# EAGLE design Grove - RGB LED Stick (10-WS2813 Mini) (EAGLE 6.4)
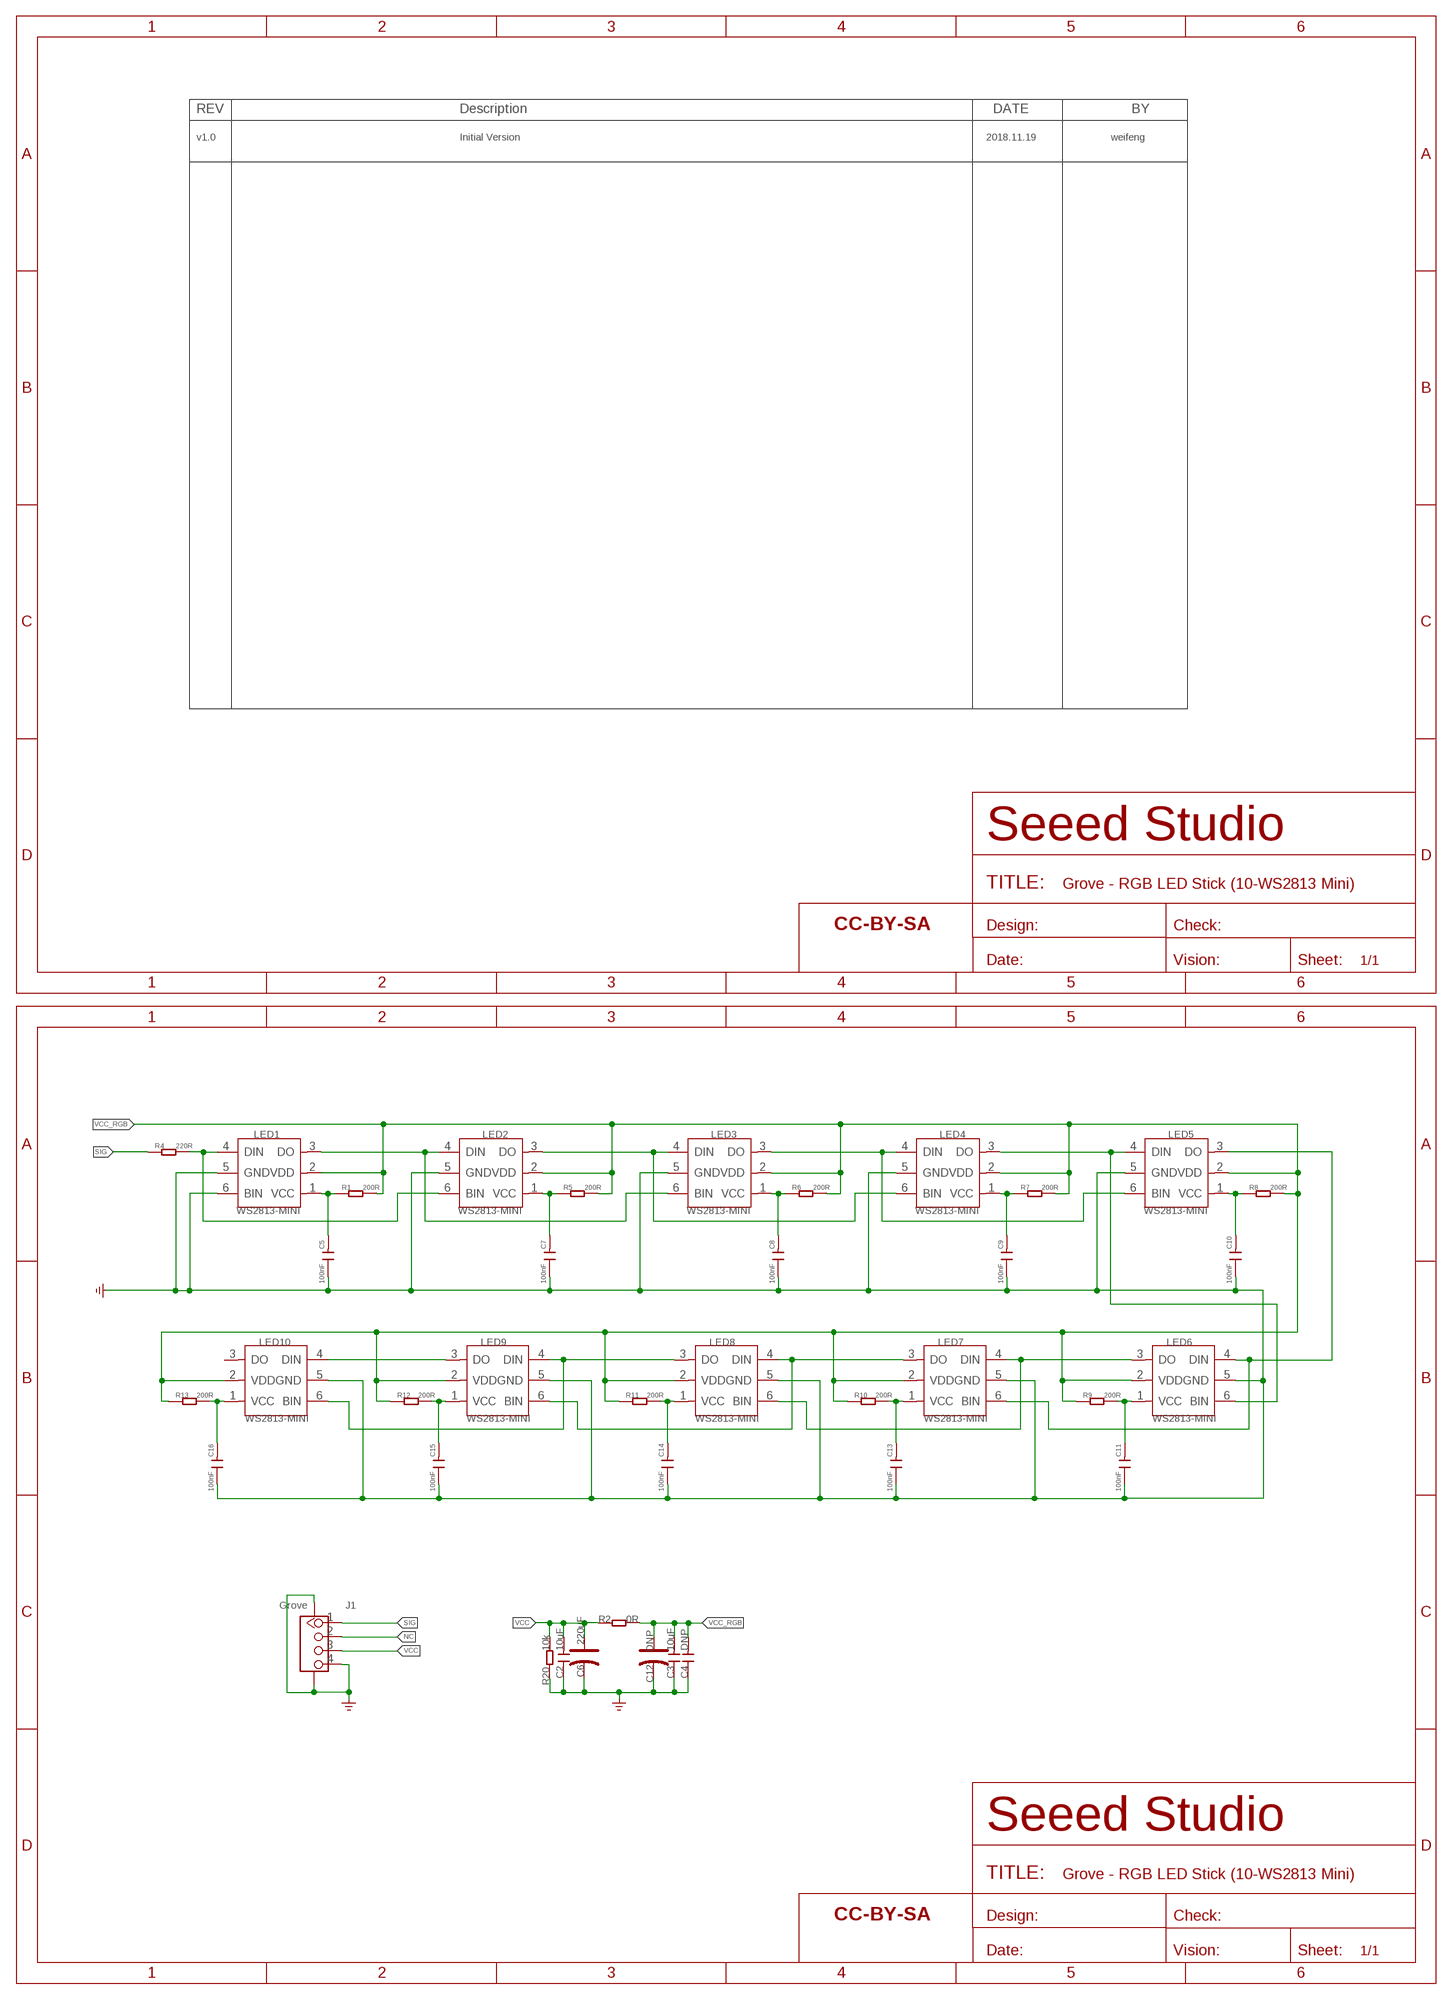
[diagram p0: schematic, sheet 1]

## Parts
C2  10uF  CAP-0805  [C0805]
C3  10uF  CAP-0805  [C0805]
C4  DNP  CAP-0603  [C0603]
C5  100nF  C-0603  [C0603]
C6  220uF  CAP-POLAR-AVX-B  [AVX-B]
C7  100nF  C-0603  [C0603]
C8  100nF  C-0603  [C0603]
C9  100nF  C-0603  [C0603]
C10  100nF  C-0603  [C0603]
C11  100nF  C-0603  [C0603]
C12  DNP  CAP-POLAR-AVX-B  [AVX-B]
C13  100nF  C-0603  [C0603]
C14  100nF  C-0603  [C0603]
C15  100nF  C-0603  [C0603]
C16  100nF  C-0603  [C0603]
FR1  SEEEDSTUDIO-OPEN-SCH-FRAME  [SEEEDSTUDIO-PCB-FRAME]
FR2  SEEEDSTUDIO-OPEN-SCH-FRAME  [SEEEDSTUDIO-PCB-FRAME]
J1  Grove  GROVE-CONNECTOR-SMD'DD'  [HW4-SMD-2.0]
LED1  WS2813-MINI  LED-RGB-6P-WS2813  [LED6-1.1-3.5X3.5X0.95MM]
LED2  WS2813-MINI  LED-RGB-6P-WS2813  [LED6-1.1-3.5X3.5X0.95MM]
LED3  WS2813-MINI  LED-RGB-6P-WS2813  [LED6-1.1-3.5X3.5X0.95MM]
LED4  WS2813-MINI  LED-RGB-6P-WS2813  [LED6-1.1-3.5X3.5X0.95MM]
LED5  WS2813-MINI  LED-RGB-6P-WS2813  [LED6-1.1-3.5X3.5X0.95MM]
LED6  WS2813-MINI  LED-RGB-6P-WS2813  [LED6-1.1-3.5X3.5X0.95MM]
LED7  WS2813-MINI  LED-RGB-6P-WS2813  [LED6-1.1-3.5X3.5X0.95MM]
LED8  WS2813-MINI  LED-RGB-6P-WS2813  [LED6-1.1-3.5X3.5X0.95MM]
LED9  WS2813-MINI  LED-RGB-6P-WS2813  [LED6-1.1-3.5X3.5X0.95MM]
LED10  WS2813-MINI  LED-RGB-6P-WS2813  [LED6-1.1-3.5X3.5X0.95MM]
R1  200R  R-0603  [R0603]
R2  0R  RES-0805  [R0805]
R4  220R  R-0603  [R0603]
R5  200R  R-0603  [R0603]
R6  200R  R-0603  [R0603]
R7  200R  R-0603  [R0603]
R8  200R  R-0603  [R0603]
R9  200R  R-0603  [R0603]
R10  200R  R-0603  [R0603]
R11  200R  R-0603  [R0603]
R12  200R  R-0603  [R0603]
R13  200R  R-0603  [R0603]
R20  10k  RES-0603  [R0603]

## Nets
GND: C2.1 C3.1 C4.1 C5.1 C6.- C7.1 C8.1 C9.1 C10.1 C11.1 C12.- C13.1 C14.1 C15.1 C16.1 J1.4 J1.SS1 J1.SS2 LED1.5(GND) LED1.6(BIN) LED2.5(GND) LED3.5(GND) LED4.5(GND) LED5.5(GND) LED6.5(GND) LED7.5(GND) LED8.5(GND) LED9.5(GND) LED10.5(GND) R20.1 ; supply symbol labelled GND_POWER
N$1: C5.2 LED1.1(VCC) R1.1
N$2: LED2.3(DO) LED3.4(DIN) LED4.6(BIN)
N$3: C9.2 LED4.1(VCC) R7.1
N$5: LED3.3(DO) LED4.4(DIN) LED5.6(BIN)
N$6: LED1.4(DIN) LED2.6(BIN) R4.2
N$7: LED4.3(DO) LED5.4(DIN) LED6.6(BIN)
N$8: C10.2 LED5.1(VCC) R8.1
N$9: LED5.3(DO) LED6.4(DIN) LED7.6(BIN)
N$10: C7.2 LED2.1(VCC) R5.1
N$12: C11.2 LED6.1(VCC) R9.2
N$14: LED1.3(DO) LED2.4(DIN) LED3.6(BIN)
N$16: C8.2 LED3.1(VCC) R6.1
N$18: LED6.3(DO) LED7.4(DIN) LED8.6(BIN)
N$21: C13.2 LED7.1(VCC) R10.2
N$23: LED7.3(DO) LED8.4(DIN) LED9.6(BIN)
N$26: C14.2 LED8.1(VCC) R11.2
N$29: LED8.3(DO) LED9.4(DIN) LED10.6(BIN)
N$32: C15.2 LED9.1(VCC) R12.2
N$35: LED9.3(DO) LED10.4(DIN)
N$38: C16.2 LED10.1(VCC) R13.2
NC: J1.2
SIG: J1.1 R4.1
VCC: C2.2 C6.+ J1.3 R2.1 R20.2
VCC_RGB: C3.2 C4.2 C12.+ LED1.2(VDD) LED2.2(VDD) LED3.2(VDD) LED4.2(VDD) LED5.2(VDD) LED6.2(VDD) LED7.2(VDD) LED8.2(VDD) LED9.2(VDD) LED10.2(VDD) R1.2 R2.2 R5.2 R6.2 R7.2 R8.2 R9.1 R10.1 R11.1 R12.1 R13.1
Unconnected: LED10.3(DO)

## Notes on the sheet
- v1.0 | Initial Version | 2018.11.19 | weifeng

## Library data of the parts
C2-C4 = Discrete-new:CAP: Ceramic Capacitors
C5 C7-C11 C13-C16 = Discrete-small:C*: Ceramic Capacitors
C6 C12 = Discrete-new:CAP-POLAR: Electrolytic Capacitors,Tantalum Capacitors and Super Capacitors
FR1 FR2 = moudle-new:SEEEDSTUDIO-OPEN-SCH-FRAME
J1 = Connector-new:GROVE-CONNECTOR-SMD: 4P-SMD-2.0:320110030;4P-SMD-2.0-90D:320110032
LED1-LED10 = Discrete-new:LED-RGB-6P
R1 R4-R13 = Discrete-small:R*
R2 R20 = Discrete-new:RES

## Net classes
3 usbvcc: width 0.203 mm, drill 0.305 mm, clearance 0.203 mm

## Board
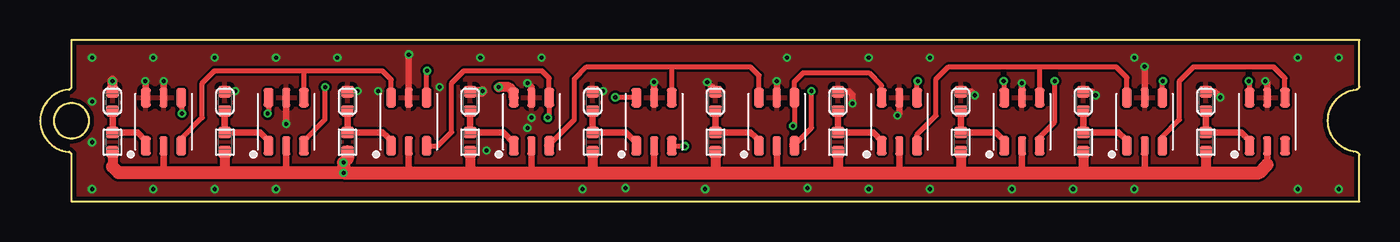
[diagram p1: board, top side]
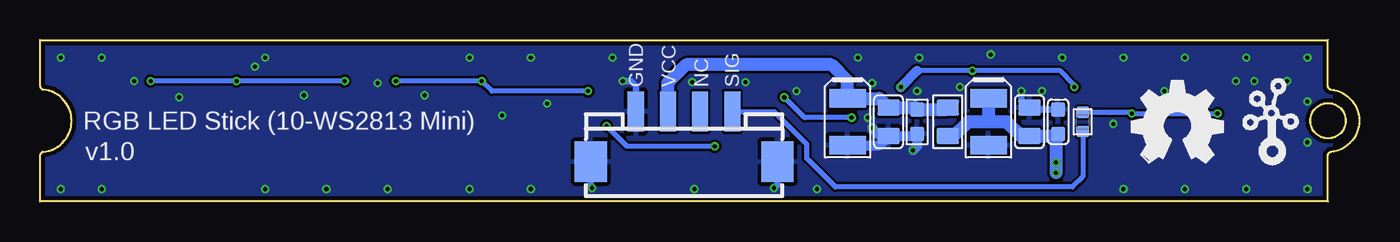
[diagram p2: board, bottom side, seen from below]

Size 81.96 x 10.03 mm. Coordinates in mm from the lower left corner, seen from the top.
Outline: 81.96,0 81.96,2.88 arc85 81.78,3.07 arc-169 81.78,6.96 arc85 81.96,7.16 81.96,10.03 1.95,10.03 1.95,7.16 arc-85 1.77,6.96 arc169 1.77,3.07 arc-85 1.95,2.88 1.95,0 81.96,0
Outline: 1.94,3.92 arc180 1.94,6.12 arc180 1.94,3.92
Copper layers (1*16): Top 0.035mm / dielectric 1.5mm / Bottom 0.035mm
Design rules "SeeedStudio_2layer_DRU_no_angle_20140221": minimum track width 1mil, minimum drill 10mil, track to track 6mil, track to pad 6mil, pad to pad 6mil, via to via 6mil, smd to smd 0mil, copper to edge 10mil, drill to drill 10mil, minimum pad ring 4mil, minimum via ring 4mil, stop-mask expansion 2mil, vias tented up to drill 25mil, thermal gap 10mil

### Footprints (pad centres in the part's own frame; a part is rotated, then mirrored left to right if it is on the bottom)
C0805 = smd 1.016 x 1.397: 1 -0.889,0; 2 0.889,0
C0603 = smd 0.889 x 0.889: 1 -0.762,0; 2 0.762,0
C0603' = smd 0.762 x 0.696: 1 0,0.602; 2 0,-0.602
AVX-B = smd 1.143 x 2.286: + 1.46,0; - -1.46,0
HW4-SMD-2.0 = smd 1 x 2.5: 1 -3,0; 2 -1,0; 3 1,0; 4 3,0 | smd 2 x 2.5: SS1 -5.8,3.123; SS2 5.8,3.123
LED6-1.1-3.5X3.5X0.95MM = smd 1.2 x 0.6: 1 -1.5,1.1; 3 -1.5,-1.1; 4 1.5,-1.1; 6 1.5,1.1 | smd 1.2 x 0.5: 2 -1.5,0; 5 1.5,0
R0603 = smd 0.762 x 0.696: 1 0,0.602; 2 0,-0.602
R0805 = smd 1.016 x 1.397: 1 -0.889,0; 2 0.889,0
R0603' = smd 0.889 x 0.889: 1 -0.762,0; 2 0.762,0

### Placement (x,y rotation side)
C2  29.25,4.95 90 bottom
C3  20.49,4.95 270 bottom
C4  18.71,4.95 270 bottom
C5  100nF  [C0603']  4.49,6.22 0 top
C6  31.79,4.95 90 bottom
C7  100nF  [C0603']  11.47,6.22 0 top
C8  100nF  [C0603']  19.09,6.22 0 top
C9  100nF  [C0603']  26.71,6.22 0 top
C10  100nF  [C0603']  34.33,6.22 0 top
C11  100nF  [C0603']  41.95,6.22 0 top
C12  23.03,4.95 90 bottom
C13  100nF  [C0603']  49.57,6.22 0 top
C14  100nF  [C0603']  57.19,6.22 0 top
C15  100nF  [C0603']  64.81,6.22 0 top
C16  100nF  [C0603']  72.43,6.22 0 top
FR1  not placed on the board
FR2  not placed on the board
J1  41.95,5.59 180 bottom
LED1  7.66,4.95 90 top
LED2  15.28,4.95 90 top
LED3  22.9,4.95 90 top
LED4  30.52,4.95 90 top
LED5  38.14,4.95 90 top
LED6  45.76,4.95 90 top
LED7  53.38,4.95 90 top
LED8  61,4.95 90 top
LED9  68.62,4.95 90 top
LED10  76.24,4.95 90 top
R1  4.49,3.68 0 top
R2  25.57,4.95 270 bottom
R4  17.19,4.95 180 bottom
R5  11.47,3.68 0 top
R6  19.09,3.68 0 top
R7  26.71,3.68 0 top
R8  34.33,3.68 0 top
R9  41.95,3.68 180 top
R10  49.57,3.68 180 top
R11  57.19,3.68 180 top
R12  64.81,3.68 180 top
R13  72.43,3.68 180 top
R20  10k  [R0603']  27.48,4.95 90 bottom
U$7  [GROVE-SILK-SMALL]  7.64,2.13 0 bottom
U$8  [OSHW_FILLX200_NOTEXT]  14.14,2.41 0 bottom

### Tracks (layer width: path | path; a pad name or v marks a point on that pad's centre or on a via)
GND  (via drill 0.25 pad 0.51)
  Top 0.406: LED1.5 v7.66,7.49 | LED1.6 6.56,7.45 v6.52,7.49 | C7.1 12.08,6.82 v12.11,6.86 | LED2.5 v15.28,4.83 | C8.1 19.7,6.82 v19.73,6.86 | LED3.5 v22.9,9.14 | LED4.5 30.52,7.11 v30.27,7.37 | C10.1 34.94,6.82 v34.97,6.86 | LED5.5 v38.14,7.43 | C11.1 41.95,6.92 v41.45,7.43 | LED6.5 v45.76,7.49 | C13.1 50.24,6.82 50.46,6.6 v50.46,6.1 | C14.1 57.86,6.82 v58.08,6.6 | LED8.5 v61,7.37 | C15.1 65.35,6.82 v65.58,6.6 | LED9.5 v68.62,8.38 | C16.1 72.97,6.82 v73.32,6.48 | LED10.5 76.24,7.37 v76.12,7.49 | LED7.5 53.38,5.46 v53.26,5.33
  Top 0.61: C5.1 v4.49,7.49 | C9.1 27.44,6.82 v27.48,6.86
  Bottom 0.406: v21,6.86 21,6.35 C3.1 20.36,5.71 C4.1 | J1.SS1 36.15,1.04 v36.37,0.82 | J1.SS2 47.75,0.91 v47.67,0.82 | J1.4 44.95,7.19 45.26,7.49 v45.76,7.49
  Bottom 0.61: v27.73,3.17 27.48,3.43 R20.1 27.6,4.06 C2.1 | C2.1 29.76,4.06 v30.27,4.57 | C6.- 29.82,3.49 C2.1
  other vias: 3.22,8.95 3.22,6.22 3.22,3.68 3.22,0.76 7.03,0.76 10.84,0.76 7.03,8.95 10.84,8.95 14.65,8.95 18.46,8.95 14.65,0.76 33.7,0.76 27.35,8.95 31.16,8.95 41.32,0.76 46.4,8.95 51.48,0.76 51.48,8.95 55.29,8.95 55.29,0.76 67.99,8.95 67.99,0.76 64.18,0.76 60.37,0.76 78.15,8.95 78.15,0.76 80.69,0.76 80.69,8.95 30.52,5.21 24.81,7.11
  pour Bottom (isolate 0.152): 1.31,10.67 82.59,10.67 82.59,-0.76 3.22,-0.76 3.22,-1.4 1.31,-1.4
  pour Top (isolate 0.152): 1.31,10.67 82.59,10.67 82.59,-0.76 1.31,-0.76
N$1
  Top 0.406: LED1.1 6.56,3.77 6.05,4.28 R1.1 C5.2
N$2  (via drill 0.25 pad 0.51)
  Top 0.305: LED3.4 24,8.08 v24.05,8.13 | LED2.3 16.38,3.77 17.7,5.08 v17.7,7.11
  Top 0.61: LED4.6 29.42,6.81 29.13,7.11 v28.49,7.11
  Bottom 0.305: v17.7,7.11 17.7,7.24 18.59,8.13 v24.05,8.13 27.48,8.13
  Bottom 0.61: 27.48,8.13 v28.49,7.11
N$3
  Top 0.406: C9.2 R7.1 28.78,4.28 29.42,3.64 LED4.1
N$5  (via drill 0.25 pad 0.51)
  Top 0.305: v31.54,5.21 31.62,5.29 LED4.4 31.62,7.66 31.16,8.13 26.33,8.13 25.57,7.37 25.57,4.32 24.71,3.45 LED3.3 | LED5.6 35.75,6.45 v35.73,6.48
  Bottom 0.305: v31.54,5.21 34.46,5.21 v35.73,6.48
N$6  (via drill 0.25 pad 0.51)
  Top 0.305: LED2.6 14.18,5.5 v14.14,5.46 | v8.81,5.46 8.81,6.41 LED1.4
  Bottom 0.305: v8.81,5.46 v14.14,5.46 14.23,5.55 R4.2
N$7
  Top 0.305: 39.29,8.38 33.95,8.38 33.19,7.62 33.19,5.08 31.62,3.51 | 39.29,8.38 44.11,8.38 44.66,7.83 LED6.6 | LED5.4 39.24,8.34 39.29,8.38
  Top 0.61: LED4.3 31.62,3.51
N$8
  Top 0.406: C10.2 R8.1 36.4,4.28 37.04,3.64 LED5.1
N$9  (via drill 0.25 pad 0.51)
  Top 0.305: LED5.3 40.02,3.45 v40.05,3.43 | v46.78,4.7 46.86,4.78 LED6.4 46.86,7.45 47.41,8 51.48,8 52.28,7.2 LED7.6
  Bottom 0.305: v40.05,3.43 45.51,3.43 v46.78,4.7
N$10
  Top 0.406: C7.2 R5.1 13.67,4.28 14.08,3.87 14.14,3.81 14.18,3.77 LED2.1
N$12
  Top 0.406: C11.2 R9.2 44.15,4.28 44.43,4 44.49,3.94 44.66,3.77 LED6.1
N$14
  Top 0.305: LED1.3 8.76,3.89 10.08,5.21 10.08,7.37 10.84,8.13 16.3,8.13 | 16.3,8.13 21.25,8.13 21.8,7.58 LED3.6 | LED2.4 16.38,8.04 16.3,8.13
N$16
  Top 0.406: C8.2 R6.1 21.29,4.28 21.57,4 21.63,3.94 21.8,3.77 LED3.1
N$18  (via drill 0.25 pad 0.51)
  Top 0.305: 46.86,3.51 47.92,4.57 v47.92,6.86 | LED7.4 54.48,7.45 v54.53,7.49 | LED8.6 59.9,7.45 v59.86,7.49
  Top 0.61: LED6.3 46.86,3.51
  Bottom 0.305: v47.92,6.86 53.89,6.86 v54.53,7.49 v59.86,7.49
N$21
  Top 0.406: C13.2 R10.2 51.77,4.28 52.28,3.77 LED7.1
N$23
  Top 0.305: LED7.3 54.48,4.15 55.67,5.33 55.67,7.62 56.43,8.38 62.02,8.38 | 62.02,8.38 66.85,8.38 67.52,7.7 LED9.6 | LED8.4 62.1,8.3 62.02,8.38
N$26
  Top 0.406: C14.2 R11.2 59.39,4.28 59.9,3.77 LED8.1
N$29  (via drill 0.25 pad 0.51)
  Top 0.305: LED8.3 62.1,4.02 63.04,4.95 v63.04,7.49 | LED9.4 69.72,7.45 v69.77,7.49 | LED10.6 75.14,7.45 v75.1,7.49
  Bottom 0.305: v63.04,7.49 v69.77,7.49 v75.1,7.49
N$32
  Top 0.406: C15.2 R12.2 67.01,4.28 67.42,3.87 67.48,3.81 67.52,3.77 LED9.1
N$35
  Top 0.305: LED9.3 69.72,4.02 70.78,5.08 70.78,7.49 71.67,8.38 76.62,8.38 77.34,7.66 LED10.4
N$38
  Top 0.406: C16.2 R13.2 74.63,4.28 75.04,3.87 75.1,3.81 75.14,3.77 LED10.1
SIG
  Bottom 0.305: R4.1 17.19,1.52 17.82,0.89 32.56,0.89 34.33,2.67 34.33,3.56 36.37,5.59 J1.1
VCC
  Bottom 0.813: J1.3 42.95,7.38 42.27,8.06 42.21,8.13 41.83,8.51 32.81,8.51 31.79,7.49 C6.+ 29.82,6.41 C2.2 27.6,5.84 R20.2 25.7,5.71 R2.1
VCC_RGB  (via drill 0.25 pad 0.51)
  Top 0.406: LED10.2 76.24,2.29 | LED1.2 7.66,1.78 | LED2.2 15.28,1.9 15.41,1.78 | LED3.2 22.9,1.9 23.03,1.78 | LED4.2 30.52,1.78 | LED5.2 38.14,1.78 | LED6.2 45.76,1.78 | LED7.2 53.38,1.78 | LED8.2 61,1.78 | LED9.2 68.62,1.9 68.75,1.78
  Top 0.61: R1.2 4.49,2.16 | R13.1 72.43,1.78 | R12.1 64.81,1.78 | R11.1 57.19,1.78 | R10.1 49.57,1.78 | R9.1 41.95,1.78 | R8.2 34.33,1.9 34.21,1.78 | R7.2 26.71,1.78 | R5.2 11.47,1.78
  Top 0.813: R6.2 19.09,2.67 v18.84,2.41 v18.84,1.78 | v18.84,1.78 15.41,1.78 11.47,1.78 7.66,1.78 4.87,1.78 4.49,2.16 | v18.84,1.78 23.03,1.78 26.71,1.78 30.52,1.78 34.21,1.78 38.14,1.78 41.95,1.78 45.76,1.78 49.57,1.78 53.38,1.78 57.19,1.78 61,1.78 64.81,1.78 68.75,1.78 72.43,1.78 75.74,1.78 76.24,2.29
  Bottom 0.813: R2.2 25.19,4.06 24.3,4.95 23.03,4.95 | 23.03,4.95 21.89,4.95 21,4.06 C3.2 18.84,4.06 | C12.+ 23.03,4.95 | 18.84,4.06 C4.2 | 18.84,4.06 v18.84,1.78

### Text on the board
bNames: SIG | NC | VCC | GND | RGB LED Stick (10-WS2813 Mini) | v1.0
